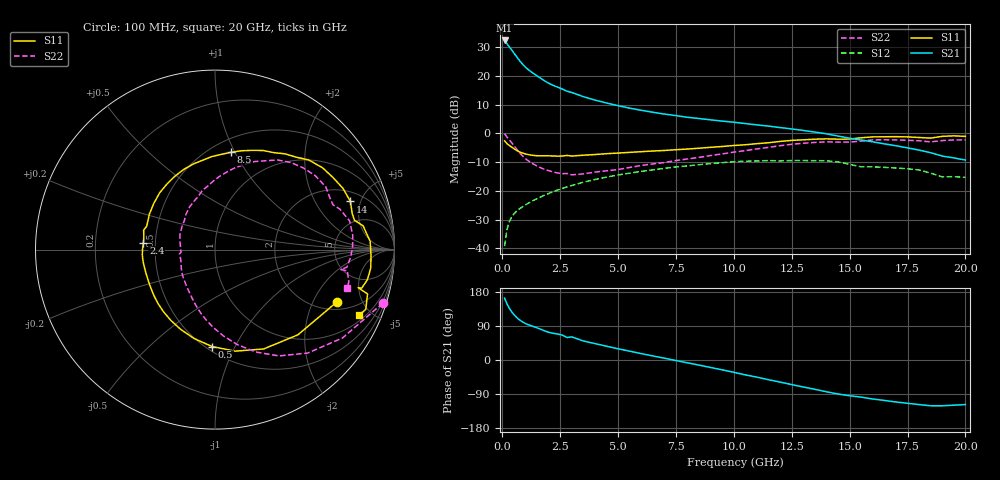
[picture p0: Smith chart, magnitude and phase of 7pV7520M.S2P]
! Infineon Technologies  Discrete & RF Semiconductors
! bfp620
! VCE = 0.75 V,  IC =  20 mA
! Common Emitter S-Parameters:  Sep 2002
# GHz  S  MA  R  50
!  f  S11  S21  S12  S22
! GHz  MAG  ANG  MAG  ANG  MAG  ANG  MAG  ANG
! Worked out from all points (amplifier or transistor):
!   59 points, 100 MHz to 20 GHz, reference 50 ohm
!   highest |S21| = 32.3 dB at 100 MHz (marker M1)
!   |S21| within 3 dB of that: start of sweep to 377.4 MHz
!   unconditionally stable (mu >= 1): 3.4 GHz to 10.19 GHz; 17.04 GHz to end of sweep
!   at 1 GHz: K = 0.69, MSG = 24.0 dB, |S12| = -24.9 dB
!   at 5.5 GHz: K = 1.04, MAG = 10.0 dB, |S12| = -13.9 dB
!   at 20 GHz: K = 1.46, MAG = -1.0 dB, |S12| = -15.3 dB
!   S11 on the Smith chart (normalised r, x): 100 MHz: 2.42, -3.11; 500 MHz: 0.53, -0.82; 2.4 GHz: 0.43, +0.04; 8.5 GHz: 0.62, +0.97; 14 GHz: 2.71, +4.05; 20 GHz: 1.28, -4.26
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0.1  0.7392 -23.2  41.13 163.2  0.0109 78.8  0.9812 -17.7
0.2  0.6624 -45.8  36.05 148.4  0.0211 68.7  0.8645 -34.7
0.3  0.6164 -63.9  32 136.9  0.0288 63.3  0.7742 -48.1
0.4  0.5768 -78.8  28.33 127.6  0.0347 59.3  0.6911 -59.0
0.5  0.5404 -91.7  24.96 120.0  0.0395 56.3  0.6133 -68.4
0.6  0.509 -103.2  21.96 113.5  0.0435 54.1  0.5434 -76.8
0.7  0.4839 -113.3  19.38 108.0  0.0471 52.6  0.4836 -84.4
0.8  0.4646 -122.1  17.25 103.4  0.0505 51.5  0.4344 -91.2
1  0.4381 -135.9  14.13 96.3  0.0569 50.5  0.3631 -102.5
1.3  0.415 -150.3  11.33 89.3  0.0665 49.9  0.2986 -115.4
1.7  0.4056 -166.0  8.82 80.1  0.0797 48.6  0.2472 -132.5
2  0.4059 -175.9  7.433 73.1  0.0898 47.2  0.2244 -145.5
2.4  0.4004 174.4  6.324 68.6  0.1034 45.0  0.2037 -157.7
3.5  0.416 151.4  4.336 50.2  0.1409 36.5  0.1968 170.4
5  0.4532 126.2  3.021 29.6  0.1886 22.7  0.2343 137.0
7  0.5028 97.8  2.16 4.8  0.2458 3.3  0.3098 107.7
8.5  0.5501 80.5  1.807 -13.5  0.2846 -12.3  0.3816 91.5
10.5  0.6321 58.7  1.476 -39.3  0.3273 -36.0  0.4999 71.1
13.5  0.7904 25.6  1.05 -77.4  0.334 -71.0  0.6939 36.4
14  0.8007 19.6  0.979 -83.8  0.3329 -77.8  0.7094 29.6
17  0.8739 -6.7  0.607 -110.7  0.249 -101.9  0.7667 0.9
20  0.8837 -24.4  0.343 -117.7  0.1712 -113.1  0.7673 -16.1
